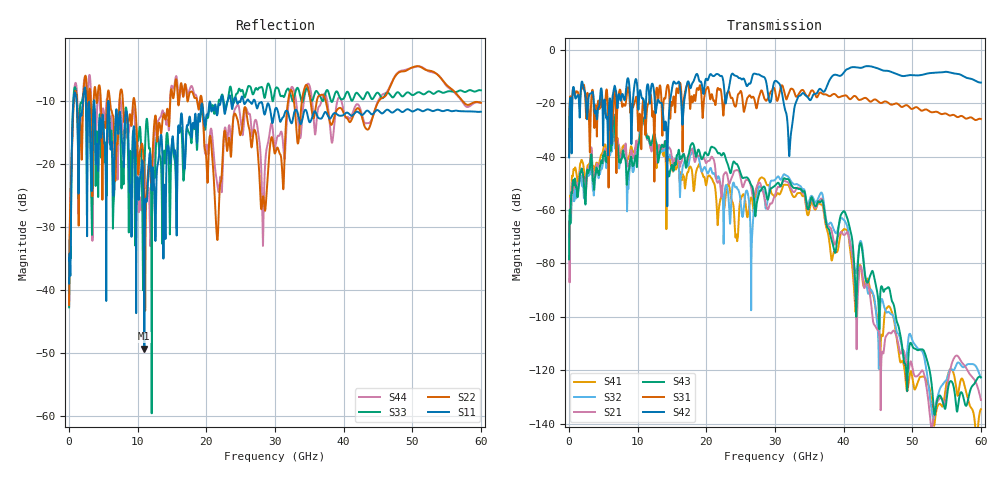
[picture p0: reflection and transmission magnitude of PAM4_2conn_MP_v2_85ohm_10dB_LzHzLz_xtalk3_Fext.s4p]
! Info: Touchstone file created by Circ.  Input file=FAB50GbE_2conn_Midplane_Examax_Topo2_v2_85ohm_10dB_LzHzLz.circ
# Hz S RI R 50
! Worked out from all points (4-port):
!   6000 points, 10 MHz to 60 GHz, reference 50 ohm
!   strongest paths, dB at 10 MHz, 15.01 GHz, 30.01 GHz, 45.01 GHz, 60 GHz:
!     S42: -40.3, -14.5, -11.7, -7.0, -12.3
!     S31: -39.8, -20.9, -15.3, -19.3, -26.0
!     S43: -78.5, -43.2, -50.9, -93.0, -122.7
!     S21: -64.6, -41.1, -54.5, -105.0, -131.2
!     S32: -69.2, -40.4, -48.7, -106.3, -122.8
!     S41: -68.5, -44.6, -55.0, -100.9, -134.6
!   lowest |S11| = -49.4 dB at 10.97 GHz (marker M1), VSWR 1.01, Z = 49.9 + j0.335 ohm
!   |S11| at or under -10 dB: 2.467 GHz to 3.616 GHz (1.149 GHz wide, 37.8 % of centre); 3.656 GHz to 22.11 GHz (18.45 GHz wide, 143 % of centre); 27.07 GHz to end of sweep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
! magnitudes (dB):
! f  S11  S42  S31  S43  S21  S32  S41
! 10 MHz  -39.0  -40.3  -39.8  -78.5  -64.6  -69.2  -68.5
! 870 MHz  -8.7  -17.7  -17.1  -48.6  -49.2  -52.2  -44.2
! 10.97 GHz  -49.4  -20.9  -22.5  -27.3  -27.4  -28.0  -26.8
! 24.4 GHz  -10.0  -9.9  -20.1  -42.7  -45.1  -51.4  -69.5
! 32.17 GHz  -13.0  -36.6  -15.2  -49.4  -51.0  -48.6  -52.0
! 41.71 GHz  -11.9  -6.6  -17.4  -88.8  -91.6  -83.2  -97.5
! 60 GHz  -11.8  -12.3  -26.0  -122.7  -131.2  -122.8  -134.6
